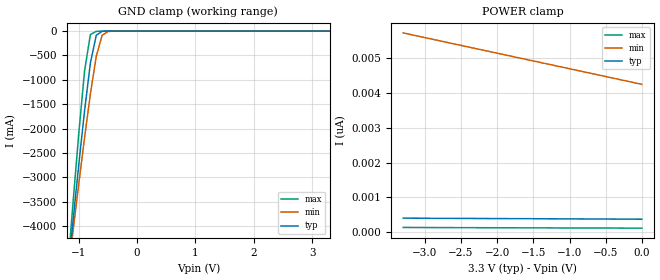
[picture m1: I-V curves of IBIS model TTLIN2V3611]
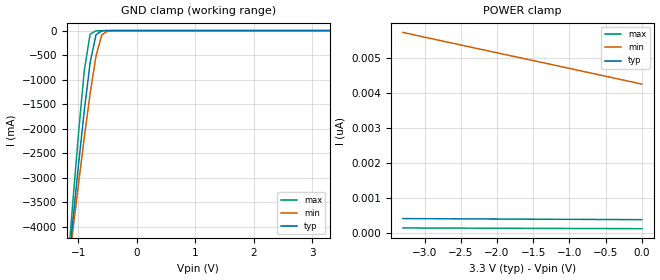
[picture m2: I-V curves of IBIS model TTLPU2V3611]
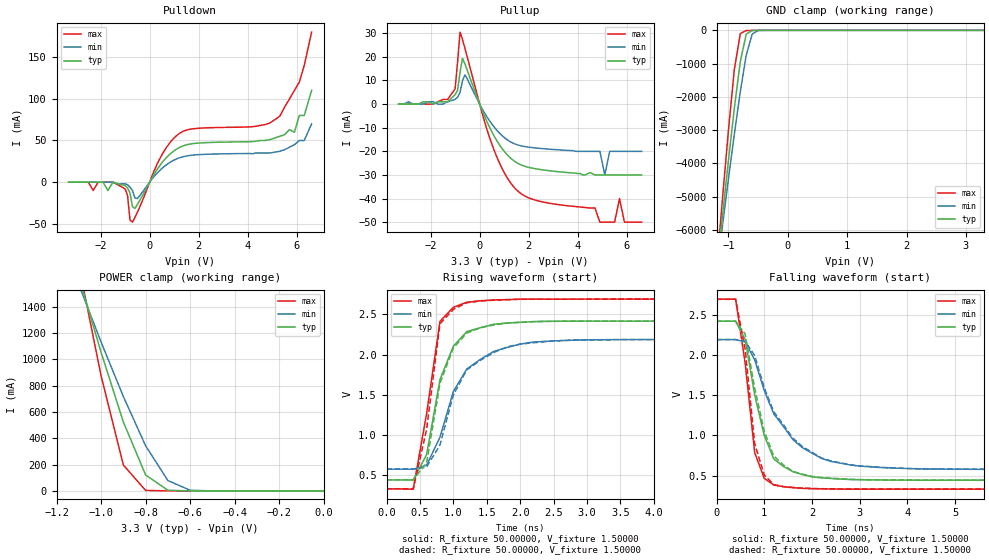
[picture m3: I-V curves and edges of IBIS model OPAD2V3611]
| IBIS file 2103bc.ibs created by s2ibis2 version 1.2
| North Carolina State University Electronics Research Laboratory  1995
[IBIS ver]   2.1
[File name]   2103bc.ibs
[File Rev]   1.0
[Date]   Friday, April 4, 2003
[Source]   IDT
[Notes]   1. Temp typ=25C, min=-40C, max=85C
   2. IDT C11_5_3.3V_SAC_2M process
   3. Ramp rates based on 50 ohm load
[Disclaimer]
READ THESE TERMS AND CONDITIONS CAREFULLY BEFORE USING THIS IBIS MODEL.  BY
USING THIS IBIS MODEL, YOU ARE ACCEPTING AND AGREEING TO THESE TERMS AND
CONDITIONS OF USE.
Integrated Device Technology, Inc. ("IDT") hereby grants the user of this
IBIS model ("User") a non-exclusive, nontransferable license to use this
IBIS model under the following terms: The User is granted this license only
to use the IBIS model for demonstration purposes only and is not granted
rights to sell, copy (except as needed to run the IBIS model), rent, lease
or sub-license (except for demonstration) the IBIS model in whole or in
part, or in modified form to anyone. The User may modify the IBIS model to
suit its specific applications, but  rights to derivative works and such
modifications shall belong to IDT.
THIS IBIS MODEL IS PROVIDED ON AN AS IS" BASIS AND IDT  MAKES ABSOLUTELY NO
WARRANTY WITH RESPECT TO THE INFORMATION CONTAINED HEREIN.  IDT DISCLAIMS
AND USER WAIVES ALL WARRANTIES, EXPRESS AND IMPLIED, INCLUDING WARRANTIES OF
MERCHANTABILITY AND FITNESS FOR A PARTICULAR PURPOSE.  THE ENTIRE RISK AS TO
QUALITY AND PERFORMANCE IS WITH THE USER  ACCORDINGLY, IN NO EVENT SHALL IDT
BE LIABLE FOR ANY DIRECT OR INDIRECT DAMAGES, WHETHER IN CONTRACT OR TORT,
INCLUDING ANY LOST PROFITS OR OTHER INCIDENTAL, CONSEQUENTIAL, EXEMPLARY, OR
PUNITIVE DAMAGES ARISING OUT OF THE USE OR APPLICATION OF THE  IBIS MODEL,
WHETHER OR NOT IDT HAD NOTICE OF SUCH DAMAGES.
IDT reserves the right to make changes without notice to any product herein
to improve reliability, function, or design. IDT does not convey any license
under patent rights or any other intellectual property rights, including
those of third parties. IDT is not obligated to provide maintenance or
support for the licensed IBIS model.
This model is for the 3.3v High-Density Supersync II 36-Bit FIFO
[Copyright]
Copyright 2002, Integrated Device Technology, Inc. All rights reserved.
|   Component 72V2103BC
[Component]   72V2103BC
[Manufacturer]   Integrated Device Technology Inc.
[Package]
|Following package parameters are for 100 lead BGA package
| variable   typ   min   max
R_pkg   82.00000m   67.00000m   0.11200
L_pkg   3.05000nH   2.45000nH   3.75000nH
C_pkg   0.36000pF   0.25000pF   0.55000pF
[Pin]  signal_name   model_name   R_pin   L_pin   C_pin
1A   WCLK   TTLIN2V3611
1B   /WEN   TTLIN2V3611
1C   /ASYW   TTLIN2V3611
1D   D17   TTLIN2V3611
1E   D16   TTLIN2V3611
1F   D13   TTLIN2V3611
1G   D11   TTLIN2V3611
1H   D8   TTLIN2V3611
1J   D6   TTLIN2V3611
1K   D5   TTLIN2V3611
2A   /PRS   TTLIN2V3611
2B   /MRS   TTLIN2V3611
2C   /SEN   TTLIN2V3611
2D   IW   TTLIN2V3611
2E   D15   TTLIN2V3611
2F   D14   TTLIN2V3611
2G   D12   TTLIN2V3611
2H   D9   TTLIN2V3611
2J   D7   TTLIN2V3611
2K   D4   TTLIN2V3611
3A   /LD   TTLIN2V3611
3B   FWFT-SI   TTLIN2V3611
3C   /FF-/IR   FLOPAD2V3611
3D   VCC   POWER
3E   VCC   POWER
3F   VCC   POWER
3G   VCC   POWER
3H   D10   TTLIN2V3611
3J   D2   TTLIN2V3611
3K   D3   TTLIN2V3611
4A   /PAF   FLOPAD2V3611
4B   OW   TTLIN2V3611
4C   VCC   POWER
4D   GND   GND
4E   GND   GND
4F   GND   GND
4G   GND   GND
4H   VCC   POWER
4J   D0   TTLIN2V3611
4K   D1   TTLIN2V3611
5A   FSEL0   TTLIN2V3611
5B   /HF   FLOPAD2V3611
5C   VCC   POWER
5D   GND   GND
5E   GND   GND
5F   GND   GND
5G   GND   GND
5H   VCC   POWER
5J   TMS   TTLPU2V3611
5K   /TRST   TTLPU2V3611
6A   /BE   TTLIN2V3611
6B   FSEL1   TTLIN2V3611
6C   VCC   POWER
6D   GND   GND
6E   GND   GND
6F   GND   GND
6G   GND   GND
6H   VCC   POWER
6J   TCK   TTLIN2V3611
6K   TDI   TTLPU2V3611
7A   /ASYR   TTLIN2V3611
7B   IP   TTLIN2V3611
7C   VCC   POWER
7D   GND   GND
7E   GND   GND
7F   GND   GND
7G   GND   GND
7H   VCC   POWER
7J   TDO   OPAD2V3611
7K   Q0   OPAD2V3611
8A   PFM   TTLIN2V3611
8B   /PAE   FLOPAD2V3611
8C   VCC   POWER
8D   VCC   POWER
8E   VCC   POWER
8F   VCC   POWER
8G   VCC   POWER
8H   Q1   OPAD2V3611
8J   Q2   OPAD2V3611
8K   Q3   OPAD2V3611
9A   RM   TTLIN2V3611
9B   /EF-/OR   FLOPAD2V3611
9C   /RT   TTLIN2V3611
9D   Q16   OPAD2V3611
9E   Q14   OPAD2V3611
9F   Q13   OPAD2V3611
9G   Q11   OPAD2V3611
9H   Q9   OPAD2V3611
9J   Q4   OPAD2V3611
9K   Q5   OPAD2V3611
10A   /REN   TTLIN2V3611
10B   RCLK   TTLIN2V3611
10C   /OE   TTLIN2V3611
10D   Q17   OPAD2V3611
10E   Q15   OPAD2V3611
10F   Q12   OPAD2V3611
10G   Q10   OPAD2V3611
10H   Q8   OPAD2V3611
10J   Q7   OPAD2V3611
10K   Q6   OPAD2V3611
| Models and submodels in the file (4): TTLIN2V3611 (Input), TTLPU2V3611 (Input), OPAD2V3611 (3-state), FLOPAD2V3611 (3-state)
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| in   in   dummy_model
| oe   oe   dummy_model
| in1  in1   dummy_model
| oe1  oe1   dummy_model
|   Model TTLIN2V3611
[Model]   TTLIN2V3611
Model_type   Input
Polarity   Non-Inverting
Vinl =  0.80000V
Vinh =  2.00000V
C_comp   10.00000pF   10.00000pF   10.00000pF
[Temperature Range]   25.00000   85.00000   -40.00000
[Voltage Range]   3.30000V   3.15000V   3.45000V
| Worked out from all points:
|   GND clamp passes 1 mA (typ) near -0.51 V on its own axis
[GND_clamp]
| voltage   I(typ)   I(min)   I(max)
-3.3V     -31.62A    -27.14A    -38.3A
-1.2V     -5.12A     -5.123A    -5.052A
-1.1V     -3.918A    -4.12A     -3.553A
-1V       -2.746A    -3.136A    -2.109A
-900mV    -1.631A    -2.183A    -811.7mA
-800mV    -652.4mA   -1.286A    -71.19mA
-700mV    -87.47mA   -520.5mA   -5.646mA
-600mV    -5.364mA   -87.77mA   -1.458mA
-500mV    -302uA     -8.09mA    -219uA
3.3V      373pA      4.31nA     115.1pA
[POWER_clamp]
| voltage   I(typ)   I(min)   I(max)
-3.3V     403.8pA    5.719nA    136.4pA
-2.6V     396.7pA    5.404nA    131.5pA
-1.3V     385pA      4.825nA    123.6pA
0V        373pA      4.243nA    116pA
|   Model TTLPU2V3611
[Model]   TTLPU2V3611
Model_type   Input
Polarity   Non-Inverting
Vinl =  0.80000V
Vinh =  2.00000V
C_comp   10.00000pF   10.00000pF   10.00000pF
[Temperature Range]   25.00000   85.00000   -40.00000
[Voltage Range]   3.30000V   3.15000V   3.45000V
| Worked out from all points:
|   GND clamp passes 1 mA (typ) near -0.51 V on its own axis
[GND_clamp]
| voltage   I(typ)   I(min)   I(max)
-3.3V     -31.62A    -27.14A    -38.3A
-1.2V     -5.12A     -5.123A    -5.052A
-1.1V     -3.918A    -4.12A     -3.553A
-1V       -2.746A    -3.136A    -2.109A
-900mV    -1.631A    -2.183A    -811.7mA
-800mV    -652.4mA   -1.286A    -71.2mA
-700mV    -87.48mA   -520.5mA   -5.659mA
-600mV    -5.37mA    -87.77mA   -1.473mA
-500mV    -314.2uA   -8.094mA   -239.3uA
3.3V      373pA      4.31nA     115.1pA
[POWER_clamp]
| voltage   I(typ)   I(min)   I(max)
-3.3V     403.8pA    5.719nA    136.4pA
-2.6V     396.7pA    5.404nA    131.5pA
-1.3V     385pA      4.825nA    123.6pA
0V        373pA      4.243nA    116pA
|   Model OPAD2V3611
[Model]   OPAD2V3611
Model_type   3-state
Polarity   Non-Inverting
Enable   Active-High
Vmeas =  1.50000V
C_comp   10.00000pF   10.00000pF   10.00000pF
[Temperature Range]   25.00000   85.00000   -40.00000
[Voltage Range]   3.30000V   3.15000V   3.45000V
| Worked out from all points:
|   slope of the pulldown table from 0 to 0.495 V, typ, clamps not added: 21.5 ohm
|   slope of the pullup table from 0 to 0.495 V, typ, clamps not added: 42.4 ohm
|   GND clamp passes 1 mA (typ) near -0.52 V on its own axis
|   POWER clamp passes 1 mA (typ) near -0.62 V on its own axis
|   rising waveform, R_fixture 50.00000, V_fixture 1.50000: 20-80 % time 343ps typ, 520ps min, 265ps max; typ from 0.444 V to 2.42 V
|   rising waveform, R_fixture 50.00000, V_fixture 1.50000: 20-80 % time 335ps typ, 490ps min, 247ps max; typ from 0.445 V to 2.42 V
|   falling waveform, R_fixture 50.00000, V_fixture 1.50000: 20-80 % time 461ps typ, 858ps min, 278ps max; typ from 2.42 V to 0.444 V
|   falling waveform, R_fixture 50.00000, V_fixture 1.50000: 20-80 % time 468ps typ, 864ps min, 295ps max; typ from 2.42 V to 0.445 V
[Pulldown]
| voltage   I(typ)   I(min)   I(max)
-3.3V     0A         0A         0A
-1V       -4mA       -2mA       -8mA
-800mV    -13.1mA    -6mA       -45.44mA
-700mV    -29.4mA    -10mA      -47.99mA
-500mV    -26.74mA   -19.63mA   -36.09mA
400mV     19.36mA    13.74mA    27.32mA
1.2V      41.38mA    29.07mA    58.2mA
5.3V      55mA       37mA       79mA
5.9V      60mA       45mA       110mA
6.1V      80mA       50mA       120mA
6.3V      80mA       50mA       140mA
6.6V      110mA      70mA       180mA
[Pullup]
| voltage   I(typ)   I(min)   I(max)
-3.3V     0A         0A         0A
-1.3V     1mA        1mA        2mA
-1V       4mA        2mA        6.5mA
-800mV    13.4mA     4.9mA      30.49mA
-600mV    17.05mA    12.41mA    23.59mA
500mV     -11.77mA   -8.469mA   -17mA
1.5V      -24.75mA   -17.12mA   -36.28mA
4.9V      -30mA      -20mA      -50mA
5.1V      -30mA      -30mA      -50mA
5.7V      -30mA      -20mA      -40mA
5.9V      -30mA      -20mA      -50mA
6.6V      -30mA      -20mA      -50mA
[GND_clamp]
| voltage   I(typ)   I(min)   I(max)
-3.3V     -44.86A    -38.5A     -54.32A
-1.2V     -7.292A    -7.294A    -7.196A
-1.1V     -5.587A    -5.872A    -5.069A
-1V       -3.924A    -4.477A    -3.02A
-900mV    -2.338A    -3.123A    -1.172A
-800mV    -940.2mA   -1.846A    -98.36mA
-700mV    -115.7mA   -749mA     -8.05mA
-600mV    -4.278mA   -114.8mA   -2.238mA
-500mV    -295.2uA   -5.816mA   -325.4uA
3.3V      607.7pA    5.602nA    92.71pA
[POWER_clamp]
| voltage   I(typ)   I(min)   I(max)
-3.3V     15.46A     11.9A      22.55A
-1.1V     1.627A     1.567A     1.714A
-1V       1.053A     1.131A     875.2mA
-900mV    523.9mA    716.9mA    196.8mA
-800mV    121.2mA    343.1mA    4.086mA
-700mV    5.031mA    78.95mA    112.4uA
-600mV    111.5uA    5.081mA    8.814uA
0V        607.7pA    2.814nA    110.2pA
[Ramp]
| variable   typ   min   max
dV/dt_r   0.80040/0.49852n   0.55518/0.74186n   1.11420/0.33285n
dV/dt_f   1.24980/0.73875n   0.95160/1.28926n   1.51836/0.39958n
R_load = 50.00000
[Rising Waveform]
R_fixture = 50.00000
V_fixture = 1.50000
V_fixture_min = 1.50000
V_fixture_max = 1.50000
| time   V(typ)   V(min)   V(max)
0s        444.1mV    577.5mV    332.7mV
400ps     443.2mV    577.5mV    329.4mV
600ps     759mV      626.9mV    1.268V
800ps     1.69V      974.8mV    2.415V
1ns       2.105V     1.542V     2.588V
1.2ns     2.286V     1.821V     2.651V
1.6ns     2.377V     2.039V     2.679V
2ns       2.402V     2.131V     2.689V
2.4ns     2.414V     2.167V     2.69V
10ns      2.417V     2.189V     2.691V
[Rising Waveform]
R_fixture = 50.00000
V_fixture = 1.50000
V_fixture_min = 1.50000
V_fixture_max = 1.50000
R_dut = 82.00000m
L_dut = 3.05000nH
C_dut = 0.36000pF
| time   V(typ)   V(min)   V(max)
0s        445.3mV    578.4mV    334.2mV
400ps     445.1mV    578.4mV    333.3mV
600ps     658.1mV    604.6mV    1.071V
800ps     1.644V     878.4mV    2.384V
1ns       2.084V     1.497V     2.563V
1.2ns     2.267V     1.81V      2.645V
1.4ns     2.333V     1.927V     2.667V
1.8ns     2.393V     2.096V     2.683V
2.6ns     2.415V     2.175V     2.689V
10ns      2.417V     2.189V     2.689V
[Falling Waveform]
R_fixture = 50.00000
V_fixture = 1.50000
V_fixture_min = 1.50000
V_fixture_max = 1.50000
| time   V(typ)   V(min)   V(max)
0s        2.417V     2.189V     2.691V
400ps     2.417V     2.189V     2.692V
600ps     2.192V     2.159V     1.896V
800ps     1.502V     1.937V     786.7mV
1ns       1V         1.557V     467.2mV
1.2ns     707.2mV    1.267V     383.9mV
1.8ns     513.6mV    846.8mV    342.6mV
2.2ns     473.3mV    714.4mV    336.7mV
2.8ns     452.6mV    633mV      333.3mV
10ns      444.1mV    577.6mV    332.7mV
[Falling Waveform]
R_fixture = 50.00000
V_fixture = 1.50000
V_fixture_min = 1.50000
V_fixture_max = 1.50000
R_dut = 82.00000m
L_dut = 3.05000nH
C_dut = 0.36000pF
| time   V(typ)   V(min)   V(max)
0s        2.417V     2.188V     2.689V
400ps     2.417V     2.188V     2.689V
600ps     2.259V     2.171V     2.07V
800ps     1.584V     1.99V      896.4mV
1ns       1.052V     1.594V     510.2mV
1.2ns     745mV      1.293V     388.5mV
1.8ns     518.7mV    861.7mV    345.7mV
2.2ns     476.7mV    720.4mV    338.7mV
2.8ns     454.5mV    636.5mV    334.8mV
10ns      445.3mV    578.4mV    334.2mV
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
